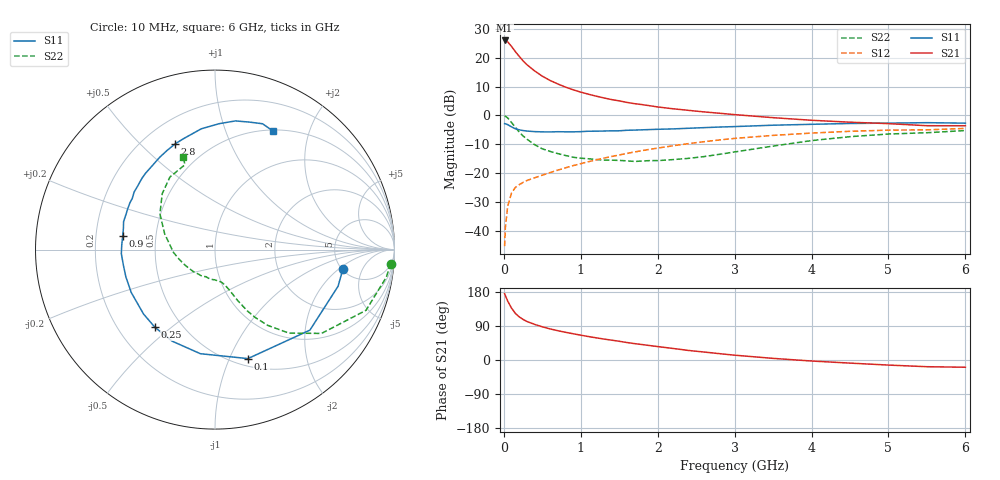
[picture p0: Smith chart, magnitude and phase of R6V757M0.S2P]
! SIEMENS Small Signal Semiconductors
! BFR193
! Si NPN RF Bipolar Junction Transistor in SOT23
! VCE = 0.75 V  IC = 7 mA
! Common Emitter S-Parameters:  May  1996
# GHz  S  MA  R  50
!  f  S11  S21  S12  S22
! GHz  MAG  ANG  MAG  ANG  MAG  ANG  MAG  ANG
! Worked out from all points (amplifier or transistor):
!   36 points, 10 MHz to 6 GHz, reference 50 ohm
!   highest |S21| = 26.0 dB at 10 MHz (marker M1)
!   |S21| within 3 dB of that: start of sweep to 125.5 MHz
!   unconditionally stable (mu >= 1): 779 MHz to 2.282 GHz
!   at 250 MHz: K = 0.54, MSG = 21.1 dB, |S12| = -23.2 dB
!   at 1.4 GHz: K = 1.06, MAG = 8.3 dB, |S12| = -14.2 dB
!   at 6 GHz: K = 0.99, MSG = 0.5 dB, |S12| = -4.5 dB
!   S11 on the Smith chart (normalised r, x): 10 MHz: 5.13, -2.28; 100 MHz: 0.58, -1.17; 250 MHz: 0.36, -0.44; 900 MHz: 0.32, +0.07; 2.8 GHz: 0.33, +0.64; 6 GHz: 0.51, +1.48
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0.01  0.7211 -8.5  20 175.1  0.0054 85.5  0.9817 -4.6
0.02  0.7154 -16.6  19.85 169.8  0.0115 79.9  0.9672 -9.1
0.05  0.6935 -40.3  18.95 155.6  0.0266 71.7  0.9069 -21.9
0.1  0.6343 -73.2  15.73 136.8  0.0452 59.4  0.7552 -38.2
0.15  0.5857 -98.0  12.79 123.0  0.0564 51.7  0.6211 -48.5
0.2  0.5633 -115.1  10.59 113.8  0.063 48.4  0.5153 -55.1
0.25  0.5472 -127.7  8.834 107.0  0.069 46.8  0.4408 -59.3
0.3  0.536 -138.0  7.597 101.7  0.0743 46.7  0.3881 -62.1
0.4  0.5243 -152.9  5.927 93.9  0.0829 48.0  0.3111 -66.0
0.5  0.5193 -163.0  4.803 87.6  0.0921 49.7  0.2637 -68.6
0.6  0.5178 -170.6  4.054 82.1  0.102 51.0  0.238 -70.5
0.7  0.5223 -177.5  3.526 77.4  0.1123 52.3  0.2183 -72.6
0.9  0.5196 171.7  2.79 69.3  0.1347 54.4  0.1885 -77.8
1.1  0.5326 163.0  2.336 61.9  0.1577 55.1  0.1772 -84.0
1.3  0.5369 154.7  2.014 55.3  0.1818 54.8  0.1682 -90.6
1.6  0.5532 144.5  1.683 46.1  0.2191 53.5  0.1632 -103.4
2.2  0.5843 126.5  1.305 30.4  0.2983 48.0  0.1715 -133.9
2.8  0.6292 110.7  1.093 16.8  0.3754 39.9  0.2114 -167.2
3.5  0.6773 96.5  0.915 4.3  0.4511 28.9  0.2943 162.5
4.5  0.7259 81.0  0.764 -8.2  0.5313 13.8  0.4286 133.3
5.5  0.7495 69.3  0.664 -17.7  0.5627 -0.8  0.5016 109.5
6  0.7355 64.0  0.663 -19.1  0.5956 -5.2  0.5473 109.0
